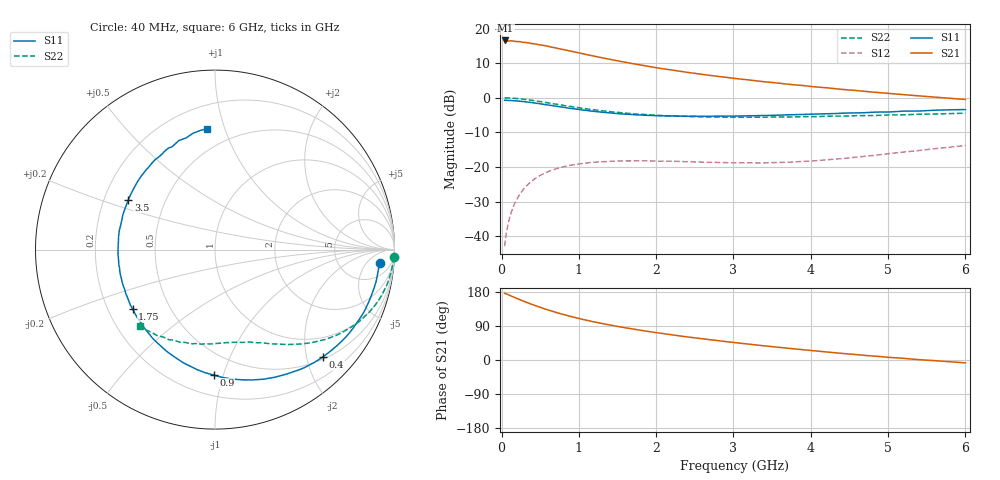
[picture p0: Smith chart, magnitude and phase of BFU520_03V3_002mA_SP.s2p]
! Filename:  P:\Prog\Test\Noise\ATS_data\Testdata_Net\03 Spar\BFU520_APG2013_37_A05_03p3V_002mA_SP_CM01_D.s2p
! Date/Time: Fri 26/Apr/2013 13:00:02
! BFU520_APG2013_37_A05_03p3V_1to20mA_SP_CM01_Bias2_R.s2p
! MDIF S-parameter v. bias file
! BFU520_APG2013_37_A05_03p3V_1to20mA_SP_CM01
! Date/time Tue Apr 23 14:11:50 2013
! VAR V_out= 3.3000
! VAR I_out= 2.0000
! VAR V_in= 0.8087
! VAR I_in= 0.0226
! Device data file deembeded for feedlines and parallel
! Original file: \03 Spar\BFU520_APG2013_37_A05_03p3V_002mA_SP_CM01_R.s2p
! Feed-files: PR047V01_250413_Feed1.s2p, PR047V01_250413_Feed2.s2p
! Parallel-file: PR047V01_250413_Par.s2p
# MHz S MA R 50
!  Freq-MHz  S11-mag  S11-arg  S21-mag  S21-arg  S12-mag  S12-arg  S22-mag  S22-arg
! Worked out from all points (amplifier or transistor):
!   98 points, 40 MHz to 6 GHz, reference 50 ohm
!   highest |S21| = 16.6 dB at 50 MHz (marker M1)
!   |S21| within 3 dB of that: start of sweep to 877 MHz
!   unconditionally stable (mu >= 1): 2.985 GHz to 5.097 GHz
!   at 300 MHz: K = 0.11, MSG = 21.0 dB, |S12| = -26.0 dB
!   at 1.6 GHz: K = 0.53, MSG = 14.3 dB, |S12| = -18.3 dB
!   at 6 GHz: K = 0.86, MSG = 6.7 dB, |S12| = -13.8 dB
!   S11 on the Smith chart (normalised r, x): 40 MHz: 12, -12; 400 MHz: 0.55, -2.32; 900 MHz: 0.34, -0.93; 1.75 GHz: 0.30, -0.29; 3.5 GHz: 0.30, +0.24; 6 GHz: 0.35, +0.87
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40  0.9198 -4.7  6.701 176.6  0.007164 87.2  0.9961 -2.4
50  0.9181 -5.8  6.723 175.1  0.008852 86.0  0.9958 -3.1
90  0.9153 -10.3  6.602 171.8  0.01589 83.6  0.9922 -5.6
120  0.9116 -13.9  6.644 169.2  0.02107 81.5  0.9879 -7.6
240  0.8892 -27.5  6.452 158.9  0.04085 73.2  0.9642 -15.0
320  0.8699 -36.3  6.281 152.4  0.05277 68.0  0.9413 -19.7
400  0.848 -44.8  6.056 146.3  0.06344 63.3  0.9142 -23.9
500  0.8174 -55.0  5.805 139.1  0.07543 57.7  0.8797 -28.8
600  0.7855 -64.8  5.552 132.2  0.08533 52.6  0.8436 -33.3
700  0.7556 -74.0  5.252 125.9  0.09351 48.1  0.8085 -37.3
900  0.6988 -90.7  4.7 114.7  0.1062 40.6  0.7461 -44.1
1050  0.6642 -102.0  4.323 107.2  0.1123 35.9  0.703 -48.5
1350  0.6105 -121.9  3.683 94.4  0.1197 28.7  0.6384 -55.6
1500  0.5906 -130.9  3.415 88.6  0.1216 25.9  0.6149 -58.7
1750  0.5652 -144.4  3.036 80.0  0.1224 22.3  0.5809 -63.4
2050  0.5499 -158.4  2.662 70.8  0.1212 19.6  0.5543 -68.6
2500  0.5411 -176.9  2.251 58.5  0.1182 18.0  0.5322 -75.9
3100  0.5453 161.7  1.855 44.1  0.1144 20.6  0.5218 -85.4
3500  0.5568 150.0  1.662 35.3  0.1154 24.2  0.5257 -91.8
4100  0.5826 133.2  1.421 23.2  0.1239 30.6  0.5346 -101.8
5200  0.6403 108.3  1.108 4.4  0.164 36.8  0.5659 -120.5
6000  0.6746 93.6  0.9458 -7.6  0.2039 35.1  0.5975 -134.5
